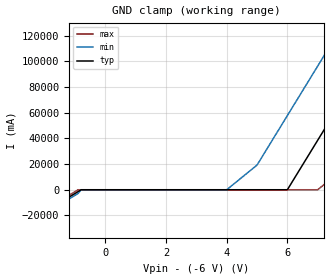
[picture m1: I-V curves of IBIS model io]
| TEXAS INSTRUMENTS INCORPORATED
| 1 Channel Uni-directional ESD-SURGE Protection Device
| Marketing Part #   Voltage Range   Package-type   #pins/pkg drawing
|   TSD03   0V-3.6V   SOD-323   2/DYF
[IBIS Ver]   4.1
[Comment char]  |_char
[File Name]   tsd03.ibs
[File Rev]   1.0
"[Date]   Jan 20, 2024 "
[Source]   Data created from TI-SPICE simulations at TI-SLL/HVL.
   The following is an IBIS list for the ESDS311.
   Please contact sllibis@ti.com with questions and
   comments concerning SLL IBIS models.
[Notes]
   - New measurements under nominal conditions only.
[Disclaimer]
"| TI and its licensors and suppliers make no warranties, either expressed"
"| or implied, with respect to this  model, including the warranties of "
"| provided solely on an ""as is"" basis. The entire risk as to its quality "
| and performance is with the customer.
[Copyright]
| (C) Copyright 2023 Texas Instruments Incorporated. All rights reserved.
| Component TSD03_DYF 2-PIN SOD-323
[Component]   TSD03_DYF
"[Manufacturer]   Texas Instruments, Inc."
[Package]   |2 SOD-323 - DYF package
   typ   min   max
R_pkg   30.0E-03   24.0E-03   36.0E-03
L_pkg   6.5E-10   5.2E-10   7.8E-10
C_pkg   5.7E-13   4.5E-13   6.8E-13
[Pin]   signal_name   model_name   R_pin   L_pin   C_pin
1   IO   io   2.07E-03   2.09E-10   6.95E-14
2   IO   io   2.07E-03   2.09E-10   6.95E-14
3   GND   gnd   2.07E-03   2.09E-10   6.95E-14
| Models and submodels in the file (1): io (Input)
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|   io Model
[Model]   io
Model_type  Input
| variable   typ   min   max
C_comp   4.5pF   3.5pF   5.5pF
[Voltage Range]   6.0   4.5   7.5
[Temperature Range]   27   -55   150
[Power Clamp Reference]   0   0   0
[GND Clamp Reference]   -6.0   -4.5   -7.5
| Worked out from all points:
|   GND clamp passes 1 mA (typ) near -0.80 V on its own axis
[GND Clamp]
|	Voltage	  I(typ)	  I(min)   I(max)
-3V       -31.4A     -32.9A     -30A
-900mV    -1.43A     -2.86A     23.8fA
-800mV    -5nA       -5nA       -5nA
4V        3.33nA     3.33nA     3.33nA
5V        4.17nA     19.2A      4.17nA
6V        5nA        57.7A      5nA
7V        38.5A      96.2A      5.83nA
8V        76.9A      135A       19.2A
9V        115A       173A       57.7A
10V       154A       212A       96.2A
11V       192A       250A       135A
30V       923A       981A       865A
[Power Clamp]
|   Voltage   I(typ)   I(min)   I(max)
-3.6V     0A         0A         0A
0V        0A         0A         0A
3.6V      0A         0A         0A
